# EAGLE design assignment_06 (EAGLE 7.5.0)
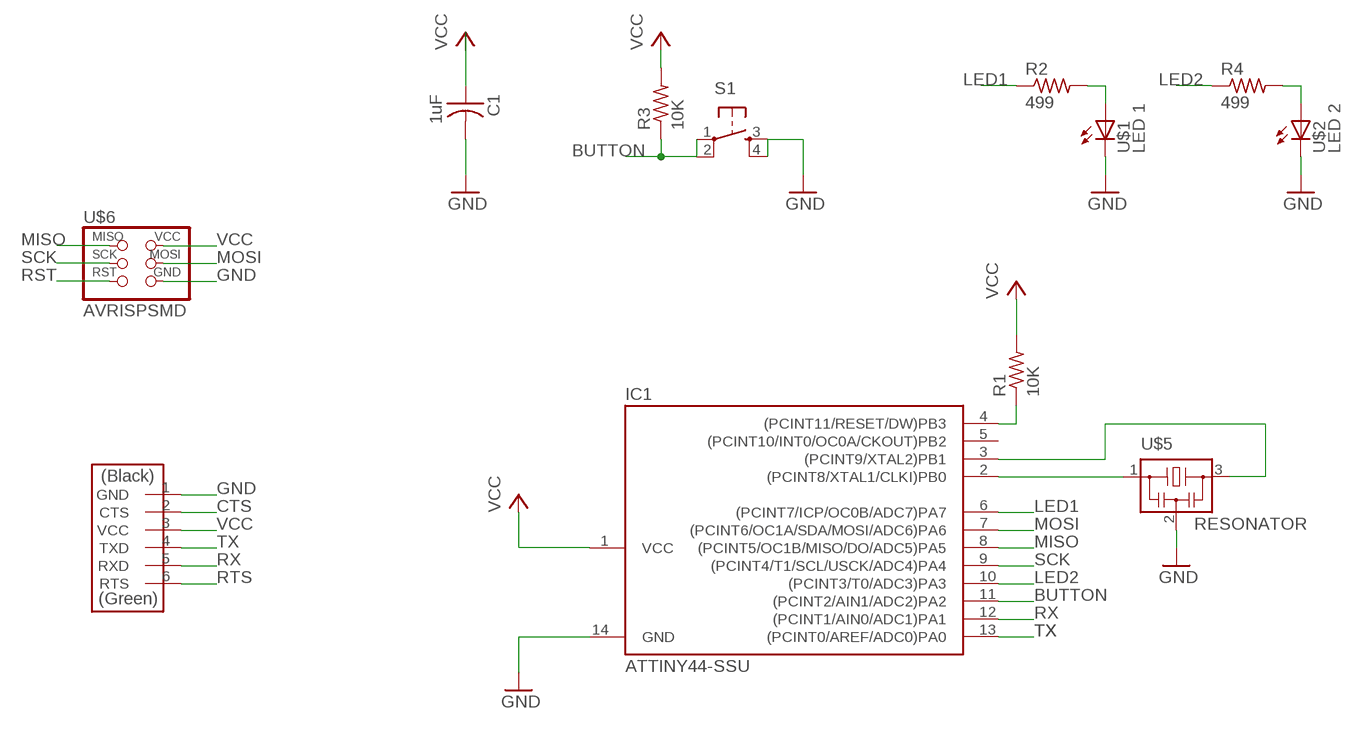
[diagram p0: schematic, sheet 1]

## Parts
C1  1uF  CAP-US1206FAB  [C1206FAB]
IC1  ATTINY44-SSU  [SOIC14]
R1  10K  RES-US1206FAB  [R1206FAB]
R2  499  RES-US1206FAB  [R1206FAB]
R3  10K  RES-US1206FAB  [R1206FAB]
R4  499  RES-US1206FAB  [R1206FAB]
S1  6MM_SWITCH6MM_SWITCH  [6MM_SWITCH]
U$1  LED 1  LEDFAB1206  [LED1206FAB]
U$2  LED 2  LEDFAB1206  [LED1206FAB]
U$4  FTDI-SMD-HEADER  [1X06SMD]
U$5  RESONATOR  [EFOBM]
U$6  AVRISPSMD  [2X03SMD]

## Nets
BUTTON: IC1.11((PCINT2/AIN1/ADC2)PA2) R3.1 S1.1(P) S1.2(P1)
CTS: U$4.2(CTS)
GND: C1.2 IC1.14(GND) S1.3(S) S1.4(S1) U$1.2(C) U$2.2(C) U$4.1(GND) U$5.2 U$6.6(GND)
LED1: IC1.6((PCINT7/ICP/OC0B/ADC7)PA7) R2.1
LED2: IC1.10((PCINT3/T0/ADC3)PA3) R4.1
MISO: IC1.8((PCINT5/OC1B/MISO/DO/ADC5)PA5) U$6.1(MISO)
MOSI: IC1.7((PCINT6/OC1A/SDA/MOSI/ADC6)PA6) U$6.4(MOSI)
N$1: R2.2 U$1.1(A)
N$2: R4.2 U$2.1(A)
N$5: IC1.2((PCINT8/XTAL1/CLKI)PB0) U$5.1
N$6: IC1.3((PCINT9/XTAL2)PB1) U$5.3
RST: IC1.4((PCINT11/RESET/DW)PB3) R1.1 U$6.5(RST)
RTS: U$4.6(RTS)
RX: IC1.12((PCINT1/AIN0/ADC1)PA1) U$4.5(RXD)
SCK: IC1.9((PCINT4/T1/SCL/USCK/ADC4)PA4) U$6.3(SCK)
TX: IC1.13((PCINT0/AREF/ADC0)PA0) U$4.4(TXD)
VCC: C1.1 IC1.1(VCC) R1.2 R3.2 U$4.3(VCC) U$6.2(VCC)
Unconnected: IC1.5((PCINT10/INT0/OC0A/CKOUT)PB2)

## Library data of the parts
C1 = fab:CAP-US
IC1 = fab:ATTINY44
R1-R4 = fab:RES-US: Resistor (US Symbol)
S1 = fab:6MM_SWITCH: OMRON SWITCH
U$1 U$2 = fab:LED: LED
U$4 = fab:FTDI-SMD-HEADER
U$5 = fab:RESONATOR
U$6 = fab:AVRISP

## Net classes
0 default: width 0.399 mm, drill 0.399 mm, clearance 0.399 mm

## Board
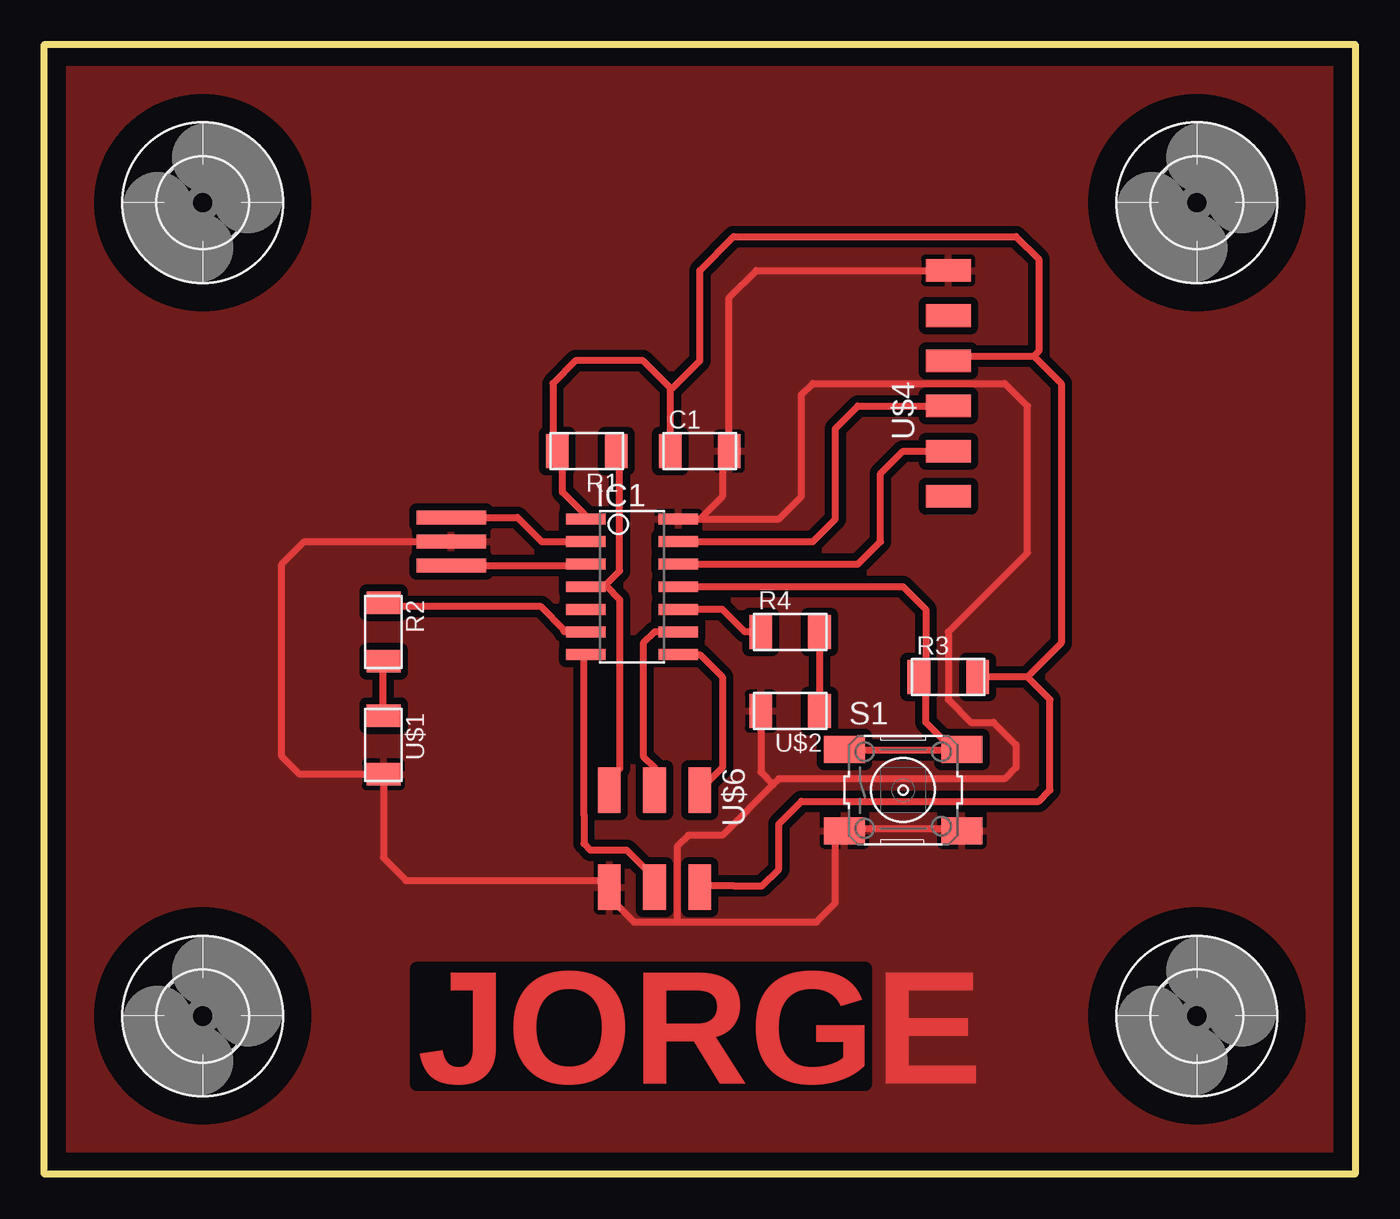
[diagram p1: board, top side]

Size 73.66 x 63.5 mm. Coordinates in mm from the lower left corner, seen from the top.
Outline: 0,63.5 73.66,63.5 73.66,0 0,0 0,63.5
Copper layers (1*16): Top 0.035mm / dielectric 1.5mm / Bottom 0.035mm
Design rules "default *": minimum track width 10mil, minimum drill 24mil, track to track 16mil, track to pad 16mil, pad to pad 16mil, via to via 16mil, smd to smd 16mil, copper to edge 40mil, drill to drill 8mil, minimum pad ring 10mil, minimum via ring 8mil, stop-mask expansion 4mil, vias tented up to drill 0mil, thermal gap 10mil

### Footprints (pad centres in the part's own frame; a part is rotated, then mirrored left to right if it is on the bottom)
C1206FAB = smd 1.27 x 1.905: 1 -1.651,0; 2 1.651,0
SOIC14 = smd 0.61 x 2.21: 1 -3.81,-2.603; 2 -2.54,-2.603; 3 -1.27,-2.603; 4 0,-2.603; 5 1.27,-2.603; 6 2.54,-2.603; 7 3.81,-2.603; 8 3.81,2.603; 9 2.54,2.603; 10 1.27,2.603; 11 0,2.603; 12 -1.27,2.603; 13 -2.54,2.603; 14 -3.81,2.603
R1206FAB = smd 1.27 x 1.905: 1 -1.651,0; 2 1.651,0
6MM_SWITCH = smd 2.286 x 1.524: 1 -3.302,2.286; 2 3.302,2.286; 3 -3.302,-2.286; 4 3.302,-2.286
LED1206FAB = smd 1.27 x 1.905: 1 -1.651,0; 2 1.651,0
1X06SMD = smd 2.54 x 1.27: 1 0,6.35; 2 0,3.81; 3 0,1.27; 4 0,-1.27; 5 0,-3.81; 6 0,-6.35
EFOBM = smd 0.8 x 3.9: 1 -1.35,0; 2 0,0; 3 1.35,0
2X03SMD = smd 2.54 x 1.27: 1 -2.54,2.54; 2 2.92,2.54; 3 -2.54,0; 4 2.92,0; 5 -2.54,-2.54; 6 2.92,-2.54
5,0 = hole 5: 0,0

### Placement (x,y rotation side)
C1  36.83,40.64 0 top
IC1  33.02,33.02 270 top
R1  30.48,40.64 180 top
R2  19.05,30.48 270 top
R3  50.8,27.94 0 top
R4  41.91,30.48 0 top
S1  48.26,21.59 0 top
U$1  19.05,24.13 270 top
U$2  41.91,26.03 180 top
U$4  50.8,44.45 0 top
U$5  22.86,35.56 270 top
U$6  34.29,19.05 270 top
U$7  [5,0]  8.89,54.61 0 top
U$8  [5,0]  64.77,54.61 0 top
U$9  [5,0]  8.89,8.89 0 top
U$10  [5,0]  64.77,8.89 0 top

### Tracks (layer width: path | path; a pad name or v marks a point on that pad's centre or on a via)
BUTTON
  Top 0.399: S1.2 51.25,23.84 45.21,23.84 S1.1
  Top 0.406: 51.25,23.84 51.09,23.84 49.53,25.4 49.53,27.56 R3.1 49.53,28.32 49.53,31.75 48.26,33.02 IC1.11
GND
  Top 0.399: 51.65,50.41 50.85,50.41 U$4.1 | S1.4 51.25,19.42 45.21,19.42 S1.3 44.81,19.01 | 37.96,14.18 35.56,14.18 33.13,14.18 31.52,15.79 U$6.6
  Top 0.406: U$6.6 31.37,16.51 20.32,16.51 19.05,17.78 U$1.2 14.35,22.48 13.33,23.49 13.33,34.29 14.6,35.56 U$5.2 | 37.96,14.18 43.39,14.18 44.45,15.24 44.45,18.8 S1.3 | U$4.1 40.01,50.8 38.48,49.28 C1.2 38.1,40.64 38.1,38.1 36.83,36.83 IC1.14 41.27,36.83 42.55,38.1 42.55,43.81 43.18,44.45 53.97,44.45 55.25,43.18 55.25,34.92 50.8,30.48 50.8,26.67 52.07,25.4 53.34,25.4 54.61,24.13 54.61,22.86 53.97,22.23 41.27,22.23 40.96,21.91 | 40.96,21.91 38.1,19.05 36.2,19.05 35.56,18.41 35.56,14.18 | U$2.2 40.26,22.61 40.96,21.91
  pour Top: 0,63.5 73.66,63.5 73.66,0 0,0
LED1
  Top 0.399: 27.9,31.9 19.45,31.9 R2.1
  Top 0.406: IC1.6 29.21,30.48 29.21,30.59 27.9,31.9
LED2
  Top 0.406: R4.1 39.37,30.48 38.1,31.75 IC1.10
MISO
  Top 0.406: IC1.8 36.83,29.21 38.1,27.94 38.1,22.86 U$6.1
MOSI
  Top 0.399: 30.31,20.22 30.31,29.08 IC1.7 | 32.33,18.21 32.73,18.21 33.94,17 33.94,16.2 U$6.4
  Top 0.406: 32.33,18.21 30.69,18.21 30.31,18.58 30.31,20.22
N$1
  Top 0.399: 19.04,25.86 U$1.1 | 19.04,28.67 R2.2
  Top 0.406: 19.04,25.86 R2.2
N$2
  Top 0.406: R4.2 U$2.1
N$5
  Top 0.406: U$5.1 26.59,36.91 27.94,35.56 IC1.2
N$6
  Top 0.406: U$5.3 30.34,34.21 IC1.3
RST
  Top 0.399: 31.52,33.1 32.33,33.91 32.33,40.35 R1.1 | 31.52,33.1 30.72,33.1 IC1.4 | 32.33,28.67 32.33,32.3 31.52,33.1 | 31.93,21.83 U$6.5
  Top 0.406: 32.33,28.67 32.33,22.8 31.75,22.23 U$6.5
RX
  Top 0.406: IC1.12 45.72,34.29 46.99,35.56 46.99,39.37 48.26,40.64 U$4.5
SCK
  Top 0.406: IC1.9 34.29,30.48 33.66,29.84 33.66,23.49 34.29,22.86 U$6.3
TX
  Top 0.406: IC1.13 43.18,35.56 44.45,36.83 44.45,41.91 45.72,43.18 U$4.4
VCC
  Top 0.399: 52.46,28.27 R3.2 52.46,27.87 | 50.85,45.99 U$4.3 | 38.77,16.2 37.16,16.2 U$6.2 | R1.2 29.11,40.35 29.11,38.34 30.31,37.13 IC1.1
  Top 0.406: 38.77,16.2 40.33,16.2 41.27,17.15 41.27,19.69 42.55,20.95 55.88,20.95 56.52,21.59 56.52,26.67 55.25,27.94 | 55.25,27.94 R3.2 | 50.85,45.99 55.61,45.99 | 55.61,45.99 57.15,44.45 57.15,29.84 55.25,27.94 | C1.1 35.18,44.2 | 35.18,44.2 33.66,45.72 29.84,45.72 28.58,44.45 28.58,40.89 R1.2 | 35.18,44.2 35.31,44.2 36.83,45.72 36.83,50.8 38.73,52.7 54.61,52.7 55.88,51.43 55.88,46.25 55.61,45.99

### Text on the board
Top: JORGE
